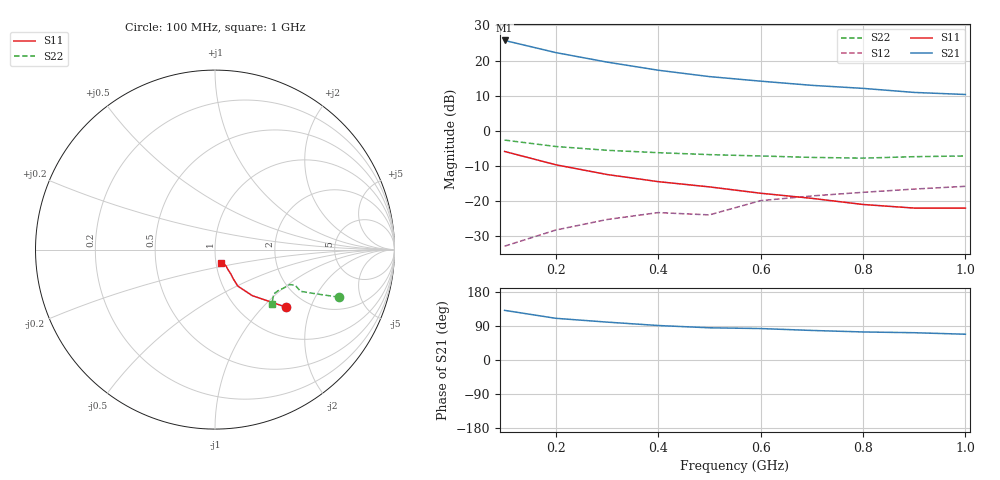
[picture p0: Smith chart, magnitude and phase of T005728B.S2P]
!AT-00572
!S-PARAMETERS at Vce=8V  Ic=20mA.  LAST UPDATED 07-21-92
# ghz s ma r 50
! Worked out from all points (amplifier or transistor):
!   10 points, 100 MHz to 1 GHz, reference 50 ohm
!   highest |S21| = 25.7 dB at 100 MHz (marker M1)
!   |S21| within 3 dB of that: start of sweep to 187 MHz
!   unconditionally stable (mu >= 1): 379.8 MHz to end of sweep
!   at 200 MHz: K = 0.84, MSG = 25.2 dB, |S12| = -28.2 dB
!   at 600 MHz: K = 1.05, MAG = 15.6 dB, |S12| = -19.8 dB
!   at 1 GHz: K = 1.03, MAG = 12.0 dB, |S12| = -15.8 dB
0.1  0.51 -39.0  19.28 131.0  0.023 77.0  0.74 -21.0
0.2  0.33 -51.0  12.96 110.0  0.039 77.0  0.6 -24.0
0.3  0.24 -58.0  9.5 100.0  0.055 77.0  0.53 -26.0
0.4  0.19 -58.0  7.28 91.0  0.069 74.0  0.49 -24.0
0.5  0.16 -57.0  5.91 85.0  0.064 72.0  0.46 -25.0
0.6  0.13 -57.0  5.09 83.0  0.102 73.0  0.44 -29.0
0.7  0.11 -56.0  4.44 78.0  0.119 70.0  0.42 -33.0
0.8  0.09 -59.0  4.02 74.0  0.134 69.0  0.41 -37.0
0.9  0.08 -64.0  3.52 72.0  0.149 70.0  0.43 -42.0
1  0.08 -64.0  3.29 68.0  0.163 68.0  0.44 -44.0
